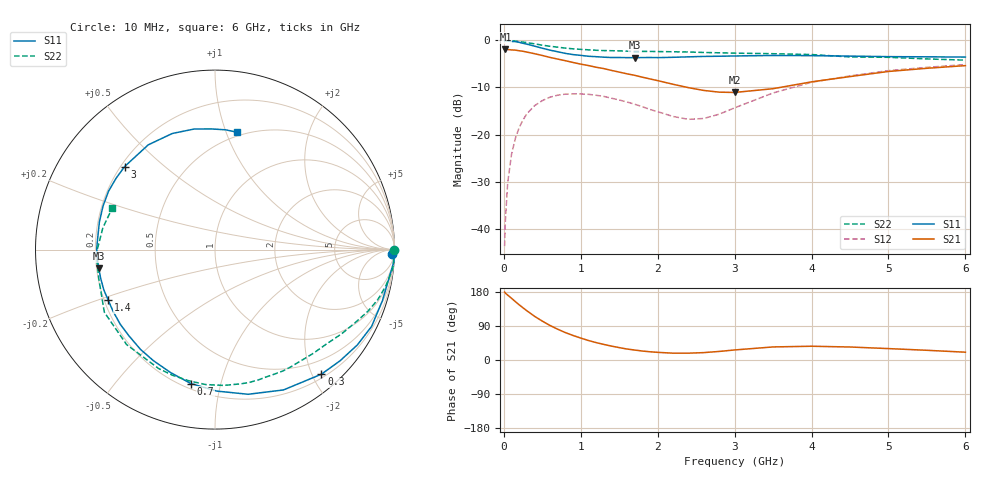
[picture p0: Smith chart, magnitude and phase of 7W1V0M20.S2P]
! Infineon Technologies  Discrete & RF Semiconductors
! BFS17W
! Si NPN RF Bipolar Junction Transistor in SOT323
! VCE = 1 V  IC = 0.2 mA
! Common Emitter S-Parameters:  August  1999
# GHz  S  MA  R  50
!  f  S11  S21  S12  S22
! GHz  MAG  ANG  MAG  ANG  MAG  ANG  MAG  ANG
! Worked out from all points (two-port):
!   36 points, 10 MHz to 6 GHz, reference 50 ohm
!   highest |S21| = -1.88 dB at 20 MHz (marker M1); lowest = -11.1 dB at 3 GHz (marker M2)
!   |S21| within 3 dB of the highest: start of sweep to 956.5 MHz
!   lowest |S11| = -3.7 dB at 1.7 GHz (marker M3), VSWR 4.81, Z = 10.5 - j3.81 ohm
!   |S11| at or under -10 dB: nowhere
!   |S22| runs from -4.2 to 0.0 dB; largest |S21 - S12| = 0.81
!   S11 on the Smith chart (normalised r, x): 10 MHz: 28, -64; 300 MHz: 0.26, -2.14; 700 MHz: 0.23, -0.81; 1.4 GHz: 0.22, -0.22; 3 GHz: 0.22, +0.37; 6 GHz: 0.46, +1.09
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0.01  0.9885 -1.5  0.798 179.1  0.0065 87.9  0.9999 -0.1
0.02  0.9999 -3.7  0.805 176.6  0.0122 86.7  0.9989 -1.2
0.05  0.9842 -8.5  0.801 171.2  0.0307 84.9  0.9973 -3.1
0.1  0.9752 -16.9  0.793 162.9  0.0617 79.2  0.9958 -6.1
0.15  0.9719 -26.1  0.789 154.0  0.0911 72.8  0.9832 -9.1
0.2  0.9546 -33.8  0.777 145.6  0.1189 68.1  0.9733 -11.8
0.3  0.9129 -49.5  0.752 129.8  0.1664 57.8  0.9488 -17.1
0.4  0.87 -64.0  0.723 115.2  0.2027 48.6  0.9196 -21.8
0.5  0.8269 -77.1  0.692 102.6  0.2292 40.7  0.8911 -25.9
0.7  0.7583 -100.2  0.634 81.2  0.262 28.1  0.8483 -33.4
0.9  0.7077 -119.0  0.583 64.7  0.2705 18.3  0.814 -40.2
1.1  0.6788 -134.9  0.541 51.4  0.2675 10.9  0.7951 -46.9
1.4  0.6585 -154.6  0.48 36.6  0.2431 3.3  0.7779 -57.2
1.7  0.6557 -170.9  0.426 26.3  0.21 0.1  0.7648 -68.1
2.2  0.6622 166.6  0.342 18.0  0.1555 9.8  0.7583 -86.3
2.6  0.6765 151.3  0.294 19.5  0.1481 31.9  0.7453 -101.3
3  0.6838 137.4  0.28 26.5  0.1921 48.2  0.7333 -115.4
3.5  0.6921 122.5  0.307 34.5  0.2766 52.1  0.7228 -133.0
4  0.6893 110.2  0.363 36.3  0.3592 47.5  0.7084 -150.5
4.5  0.6818 99.7  0.413 34.3  0.4197 41.1  0.6676 -165.9
5.5  0.67 84.9  0.506 25.6  0.5177 28.8  0.6363 168.9
6  0.6654 79.6  0.54 20.6  0.5545 23.1  0.6173 157.9
